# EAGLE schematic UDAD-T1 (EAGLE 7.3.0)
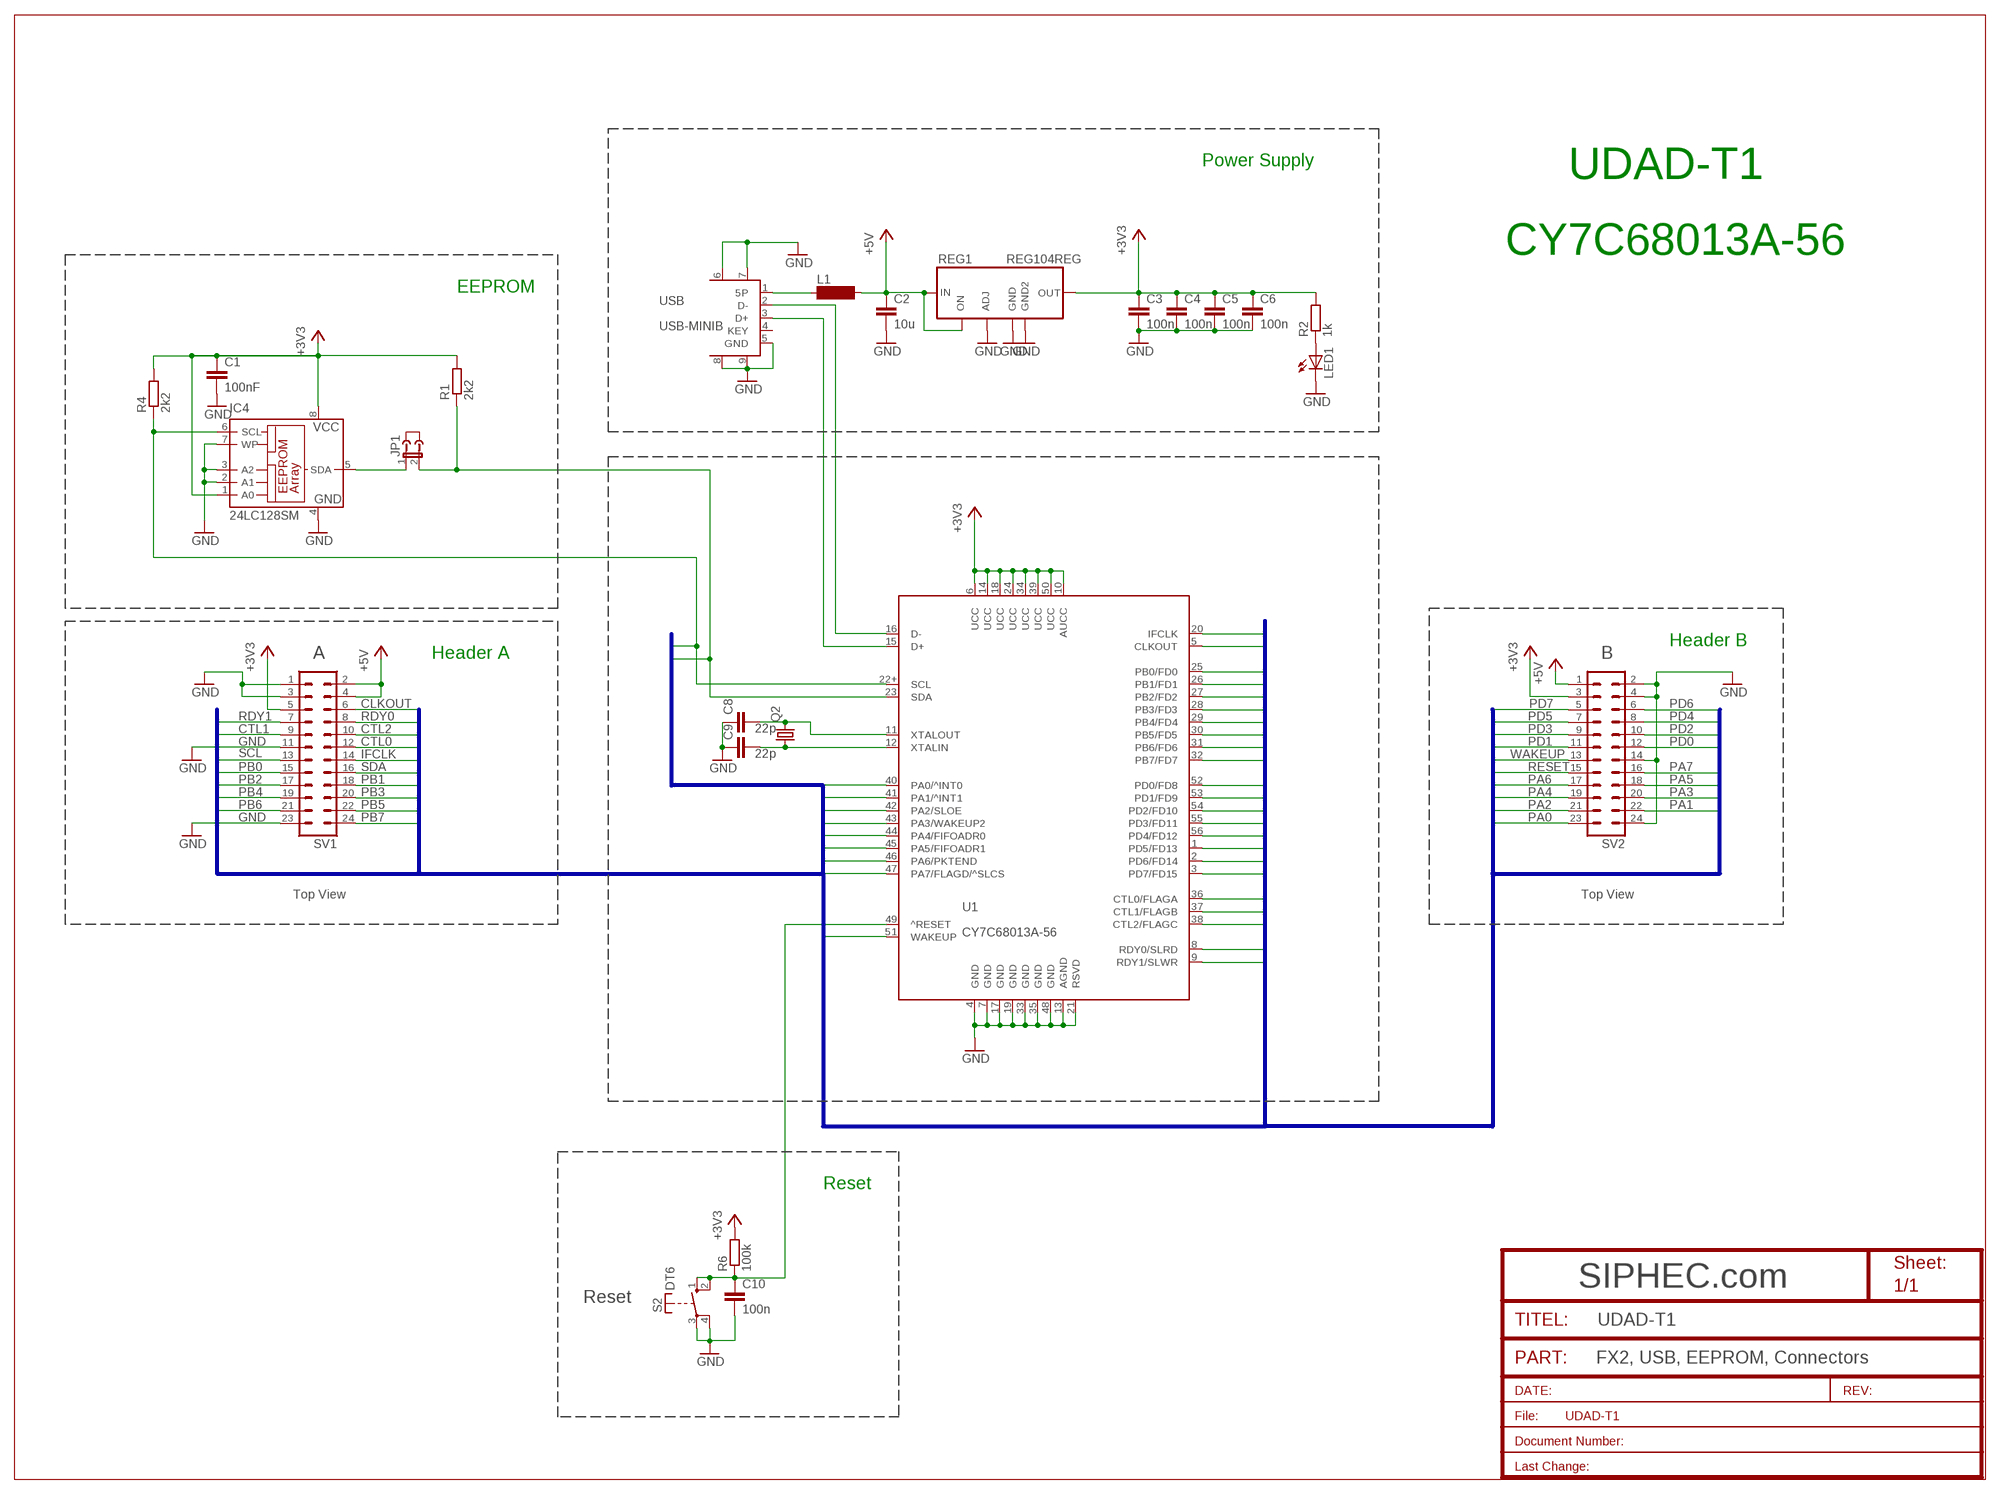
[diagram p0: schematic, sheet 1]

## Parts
C1  100nF  C-EUC0805  [C0805]
C2  10u  C-EUC0805  [C0805]
C3  100n  C-EUC0805  [C0805]
C4  100n  C-EUC0805  [C0805]
C5  100n  C-EUC0805  [C0805]
C6  100n  C-EUC0805  [C0805]
C8  22p  C-EUC1206  [C1206]
C9  22p  C-EUC1206  [C1206]
C10  100n  C-EUC1206  [C1206]
IC4  24LC128SM  24LC64SM  [SO-08M]
J1  JUMPER  [JUMP]
JP1  JP1E  [JP1]
L1  SM-Z15  [SM-Z15]
LED1  LEDCHIPLED_0805  [CHIPLED_0805]
Q2  CRYTALHC49U-V  [HC49U-V]
R1  2k2  R-EU_M1206  [M1206]
R2  1k  R-EU_M1206  [M1206]
R4  2k2  R-EU_M1206  [M1206]
R6  100k  R-EU_M1206  [M1206]
REG1  REG104REG  [SOT223-5]
S2  DT6  [DT6]
SV1  MA12-2  [MA12-2]
SV2  MA12-2  [MA12-2]
U1  CY7C68013A-56  CY7C68013-56PVC  [SSOP56]
USB  USB-MINIB  USB-MINIB-BO_NO_HOLES  [USB-MINIB-BO_NO_HOLES]

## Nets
5P: L1.1 USB.1(5P)
+3V3: C1.1 C3.1 C4.1 C5.1 C6.1 IC4.1(A0) IC4.8(VCC) R1.2 R2.2 R4.2 R6.2 REG1.2(OUT) SV1.5 SV2.3 U1.6(UCC) U1.10(AUCC) U1.14(UCC) U1.18(UCC) U1.24(UCC) U1.34(UCC) U1.39(UCC) U1.50(UCC)
+5V: C2.1 L1.2 REG1.1(IN) REG1.5(EN) SV1.2 SV1.4 SV2.1
CLKOUT: SV1.6 U1.5(CLKOUT)
CTL0: SV1.12 U1.36(CTL0/FLAGA)
CTL1: SV1.9 U1.37(CTL1/FLAGB)
CTL2: SV1.10 U1.38(CTL2/FLAGC)
GND: C1.2 C2.2 C3.2 C4.2 C5.2 C6.2 C8.1 C9.1 C10.2 IC4.2(A1) IC4.3(A2) IC4.4(GND) IC4.7(WP) LED1.C REG1.3(GND) REG1.4(ADJ) REG1.6(GND2) S2.3(P) S2.4(P) SV1.1 SV1.3 SV1.11 SV1.23 SV2.2 SV2.4 SV2.14 SV2.24 U1.4(GND) U1.7(GND) U1.13(AGND) U1.17(GND) U1.19(GND) U1.21(RSVD) U1.33(GND) U1.35(GND) U1.48(GND) USB.5(GND) USB.6(GND) USB.7(GND) USB.8(GND) USB.9(GND)
IFCLK: SV1.14 U1.20(IFCLK)
N$2: IC4.5(SDA) JP1.1
N$4: LED1.A R2.1
N$15: U1.16(D-) USB.2(D-)
N$16: U1.15(D+) USB.3(D+)
N$36: C9.2 Q2.1 U1.12(XTALIN)
N$37: C8.2 Q2.2 U1.11(XTALOUT)
PA0: SV2.23 U1.40(PA0/^INT0)
PA1: SV2.22 U1.41(PA1/^INT1)
PA2: SV2.21 U1.42(PA2/SLOE)
PA3: SV2.20 U1.43(PA3/WAKEUP2)
PA4: SV2.19 U1.44(PA4/FIFOADR0)
PA5: SV2.18 U1.45(PA5/FIFOADR1)
PA6: SV2.17 U1.46(PA6/PKTEND)
PA7: SV2.16 U1.47(PA7/FLAGD/^SLCS)
PB0: SV1.15 U1.25(PB0/FD0)
PB1: SV1.18 U1.26(PB1/FD1)
PB2: SV1.17 U1.27(PB2/FD2)
PB3: SV1.20 U1.28(PB3/FD3)
PB4: SV1.19 U1.29(PB4/FD4)
PB5: SV1.22 U1.30(PB5/FD5)
PB6: SV1.21 U1.31(PB6/FD6)
PB7: SV1.24 U1.32(PB7/FD7)
PD0: SV2.12 U1.52(PD0/FD8)
PD1: SV2.11 U1.53(PD1/FD9)
PD2: SV2.10 U1.54(PD2/FD10)
PD3: SV2.9 U1.55(PD3/FD11)
PD4: SV2.8 U1.56(PD4/FD12)
PD5: SV2.7 U1.1(PD5/FD13)
PD6: SV2.6 U1.2(PD6/FD14)
PD7: SV2.5 U1.3(PD7/FD15)
RDY0: SV1.8 U1.8(RDY0/SLRD)
RDY1: SV1.7 U1.9(RDY1/SLWR)
RESET: C10.1 R6.1 S2.1(S) S2.2(S) SV2.15 U1.49(^RESET)
SCL: IC4.6(SCL) R4.1 SV1.13 U1.22+(SCL)
SDA: JP1.2 R1.1 SV1.16 U1.23(SDA)
WAKEUP: SV2.13 U1.51(WAKEUP)
Unconnected: USB.4(KEY)

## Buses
CLKOUT,IFCLK,RDY0,RDY1,CTL0,CTL1,CTL2,PA[0..7],PB[0..7],PD[0..7],SCL,SDA,WAKEUP,RESET

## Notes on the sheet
- Power Supply
- UDAD-T1
- CY7C68013A-56
- EEPROM
- Header B
- A | Header A | B
- Top View | Top View
- Reset
- Reset
- UDAD-T1
- FX2, USB, EEPROM, Connectors

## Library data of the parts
C1-C6 = my_lbr:C-EU: CAPACITOR, European symbol
C8-C10 = rcl:C-EU: CAPACITOR, European symbol
IC4 = microchip:24*: Serial EEPROM I2C
J1 = jumper:JUMPER: JUMPER header
JP1 = jumper:JP1E: JUMPER
L1 = inductor-neosid:SM-Z15: INDUCTOR
LED1 = led:LED: LED
Q2 = crystal:CRYTAL: CRYSTAL
R1 R2 R4 R6 = rcl:R-EU_: RESISTOR, European symbol
REG1 = my_lbr:REG104
S2 = switch-misc:DT: ITT SWITCH
SV1 SV2 = con-lstb:MA12-2: PIN HEADER
U1 = my_lbr:CY7C68013-56: FX2
USB = my_lbr:USB-MINIB-BO_NO_HOLES: USB MiniB-Buchse Oberflächenmontage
